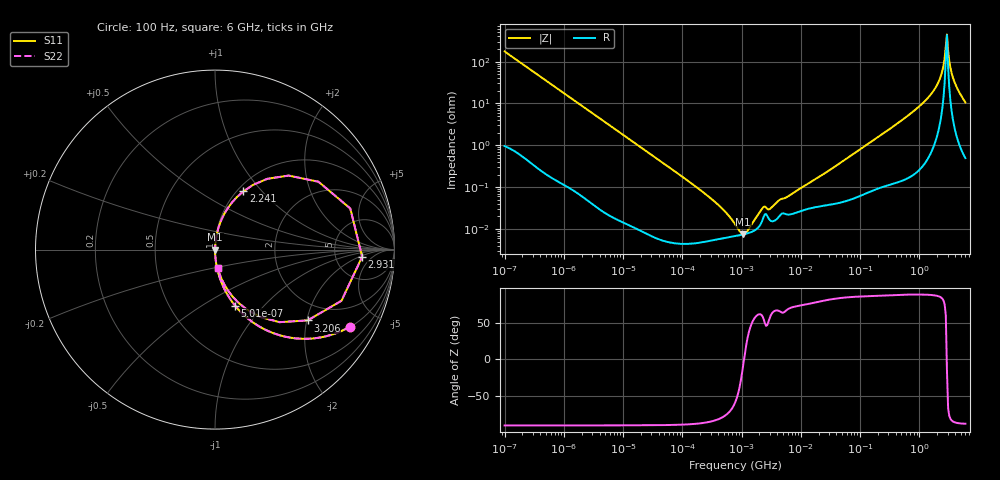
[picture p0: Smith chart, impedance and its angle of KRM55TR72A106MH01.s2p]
!Murata Part Number: KRM55TR72A106MH01
!These Parameters are Measured in Series Mode Connection
!Data Generated on Jan 08, 2026
!  o--ll--o
!Port1  Port2
!  o------o
!Operation Temp=25[degC], DC Bias Voltage=0[V]
!Freq. Start=100[Hz] Stop=6[GHz] 401[Steps]
# Hz S RI R 50
!Freq.(Hz) S11(Real) S11(Imag) S21(Real) S21(Imag) S12(Real) S12(Imag) S22(Real) S22(Imag)
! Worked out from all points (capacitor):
!   401 points, 100 Hz to 6 GHz, reference 50 ohm
!   read as one part in series: C = 9.07 uF near 109 Hz
!   lowest |Z| = 7.5 mohm at 1.06 MHz (marker M1)
!   series resonance near 1.099 MHz, so ESL is about 2.3 nH
!   S11 on the Smith chart (normalised r, x): 100 Hz: 1.02, -3.50; 501 Hz: 1.00, -0.70; 2.241 GHz: 1.07, +0.80; 2.931 GHz: 9.58, -2.36; 3.206 GHz: 1.48, -2.02; 6 GHz: 1.01, -0.21
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100  0.7529 -0.4286  0.2471 0.4286  0.2471 0.4286  0.7529 -0.4286
205  0.4247 -0.4912  0.5753 0.4912  0.5753 0.4912  0.4247 -0.4912
501  0.1115 -0.3119  0.8885 0.3119  0.8885 0.3119  0.1115 -0.3119
2008  0.00833 -0.0875  0.9917 0.0875  0.9917 0.0875  0.00833 -0.0875
40335  7.64e-05 -0.00444  0.9999 0.00444  0.9999 0.00444  7.64e-05 -0.00444
316350  5.37e-05 -0.000509  0.9999 0.000509  0.9999 0.000509  5.37e-05 -0.000509
774597  6.8e-05 -0.000113  0.9999 0.000113  0.9999 0.000113  6.8e-05 -0.000113
1059725  7.41e-05 -1.15e-05  0.9999 1.15e-05  0.9999 1.15e-05  7.41e-05 -1.15e-05
1386327  8.24e-05 7.53e-05  0.9999 -7.53e-05  0.9999 -7.53e-05  8.24e-05 7.53e-05
2268635  0.000167 0.00027  0.9998 -0.00027  0.9998 -0.00027  0.000167 0.00027
3103719  0.000157 0.000271  0.9998 -0.000271  0.9998 -0.000271  0.000157 0.000271
1.555665e7  0.000322 0.00135  0.9997 -0.00135  0.9997 -0.00135  0.000322 0.00135
3.124326e8  0.00172 0.0242  0.9983 -0.0242  0.9983 -0.0242  0.00172 0.0242
1.197065e9  0.0149 0.1061  0.9851 -0.1061  0.9851 -0.1061  0.0149 0.1061
2.240541e9  0.158 0.3245  0.842 -0.3245  0.842 -0.3245  0.158 0.3245
2.562649e9  0.4102 0.4125  0.5898 -0.4125  0.5898 -0.4125  0.4102 0.4125
2.679998e9  0.5766 0.378  0.4234 -0.378  0.4234 -0.378  0.5766 0.378
2.931063e9  0.8199 -0.0401  0.1801 0.0401  0.1801 0.0401  0.8199 -0.0401
3.205649e9  0.5162 -0.3944  0.4838 0.3944  0.4838 0.3944  0.5162 -0.3944
3.505958e9  0.2506 -0.3748  0.7494 0.3748  0.7494 0.3748  0.2506 -0.3748
4.009986e9  0.1001 -0.2641  0.8999 0.2641  0.8999 0.2641  0.1001 -0.2641
6e9  0.0157 -0.1032  0.9843 0.1032  0.9843 0.1032  0.0157 -0.1032
